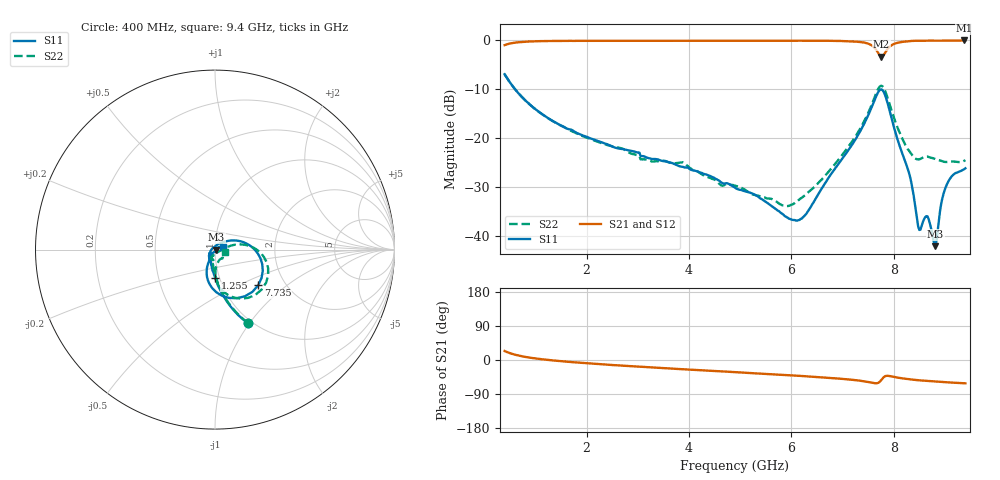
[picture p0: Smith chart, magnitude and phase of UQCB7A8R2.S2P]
!  Part Number  UQCB7A8R2	Mounting Orientation: Vertical
!  Description: RF capacitors
!  Application: Coupling, Bypass, Tuning, DC Block
!  Filters, Matching
# GHZ S DB R 50
! Freq  |S11|  S11 Ph  |S21|  S21 Ph  |S12|  S12 Ph  |S22|  S22 Ph
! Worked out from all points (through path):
!   401 points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, 400 MHz to 9.4 GHz, reference 50 ohm
!   highest |S21| = -0.05 dB at 9.378 GHz (marker M1); lowest = -3.4 dB at 7.758 GHz (marker M2)
!   group delay of S21, straight-line fit = 21.9 ps
!   lowest |S11| = -42.1 dB at 8.815 GHz (marker M3), VSWR 1.02, Z = 50.8 - j0.0491 ohm
!   |S11| at or under -10 dB: 602.2 MHz to end of sweep
!   |S22| runs from -33.9 to -7.0 dB; largest |S21 - S12| = 0.0014
!   S11 on the Smith chart (normalised r, x): 400 MHz: 0.95, -0.98; 1.255 GHz: 0.95, -0.31; 7.735 GHz: 1.46, -0.65; 9.4 GHz: 1.10, +0.03
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0.4  -6.96 -66.0  -1.01 23.7  -1.01 23.8  -6.97 -65.7
1.255  -15.97 -89.6  -0.16 0.1  -0.17 0.1  -16.01 -87.7
1.908  -19.41 -98.4  -0.12 -7.6  -0.12 -7.6  -19.53 -94.1
3.415  -24.47 -119.3  -0.11 -20.7  -0.11 -20.6  -24.80 -100.6
3.888  -25.91 -130.3  -0.14 -24.5  -0.14 -24.4  -25.00 -109.6
4.9  -30.15 -150.8  -0.11 -32.0  -0.11 -32.0  -29.75 -100.6
6.048  -36.77 122.8  -0.11 -40.9  -0.11 -40.9  -33.44 -38.7
6.408  -33.57 79.0  -0.10 -44.0  -0.10 -44.0  -30.42 -12.1
7.083  -22.95 38.9  -0.20 -50.8  -0.19 -50.8  -22.24 13.1
7.465  -16.17 16.6  -0.59 -57.3  -0.58 -57.2  -15.69 9.6
7.623  -12.34 -5.9  -1.52 -61.3  -1.52 -61.3  -11.77 -4.8
7.735  -10.11 -39.6  -3.20 -56.2  -3.20 -56.2  -9.39 -32.9
7.758  -10.05 -48.5  -3.36 -52.6  -3.36 -52.6  -9.31 -40.5
7.915  -14.21 -99.0  -1.38 -42.2  -1.37 -42.2  -12.94 -80.9
8.298  -27.10 -123.0  -0.21 -50.6  -0.20 -50.6  -22.59 -77.8
8.478  -38.11 -101.6  -0.13 -53.4  -0.12 -53.4  -24.39 -58.7
8.658  -36.00 -53.1  -0.10 -55.3  -0.09 -55.3  -23.79 -49.3
8.815  -42.12 -3.5  -0.10 -57.0  -0.09 -57.0  -24.32 -44.8
8.95  -32.33 33.4  -0.11 -58.2  -0.10 -58.2  -24.74 -38.7
9.04  -29.45 27.6  -0.11 -58.9  -0.10 -58.9  -24.90 -33.6
9.378  -26.37 16.8  -0.05 -61.4  -0.05 -61.4  -24.67 -16.2
9.4  -26.19 17.1  -0.05 -61.6  -0.04 -61.5  -24.53 -15.0
